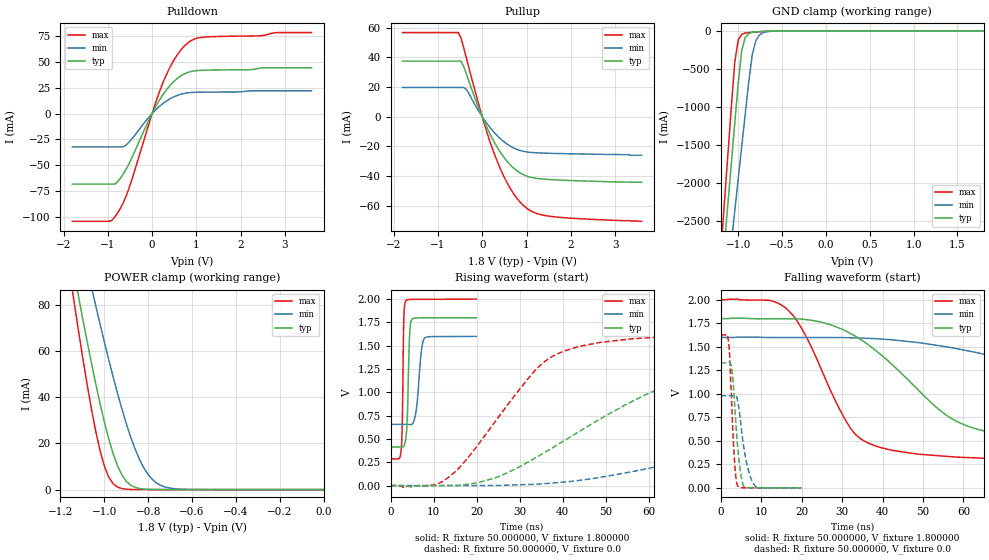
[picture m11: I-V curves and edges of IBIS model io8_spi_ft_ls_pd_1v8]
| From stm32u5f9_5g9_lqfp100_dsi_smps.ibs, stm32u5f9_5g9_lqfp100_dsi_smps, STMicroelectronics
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|   Model io8_spi_ft_ls_pd_1v8
[Model]  io8_spi_ft_ls_pd_1v8
Model_type I/O
Polarity   Non-Inverting
Enable   Active-Low
Vinl =   0.540000V
Vinh =   1.260000V
Vmeas =  0.900000V
Cref =   50.000000pF
Rref =   100.000000M
Vref =   0.0V
C_comp   3.338500pF   3.332300pF   3.378900pF
[Temperature Range]   25.000000   0.140000k   -40.000000
[Pullup Reference]   1.800000V   1.600000V   2.000000V
[Pulldown Reference]   0.0V   0.0V   0.0V
[POWER Clamp Reference]   1.800000V   1.600000V   2.000000V
[GND Clamp Reference]   0.0V   0.0V   0.0V
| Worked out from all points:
|   slope of the pulldown table from 0 to 0.27 V, typ, clamps not added: 13.6 ohm
|   slope of the pullup table from 0 to 0.27 V, typ, clamps not added: 15.9 ohm
|   GND clamp passes 1 mA (typ) near -0.50 V on its own axis
|   POWER clamp passes 1 mA (typ) near -0.86 V on its own axis
|   rising waveform, R_fixture 50.000000, V_fixture 1.800000: 20-80 % time 490ps typ, 1.02ns min, 316ps max; typ from 0.414 V to 1.8 V
|   rising waveform, R_fixture 50.000000, V_fixture 0.0: 20-80 % time 31.5ns typ, 69.2ns min, 16.6ns max; typ from 0 V to 1.33 V
|   falling waveform, R_fixture 50.000000, V_fixture 1.800000: 20-80 % time 22.7ns typ, 57.7ns min, 11.6ns max; typ from 1.8 V to 0.414 V
|   falling waveform, R_fixture 50.000000, V_fixture 0.0: 20-80 % time 1.42ns typ, 2.11ns min, 1.03ns max; typ from 1.33 V to 0 V
[Pulldown]
|Voltage   I(typ)   I(min)   I(max)
-1.8V     -68.38mA   -32.32mA   -104.4mA
-960mV    -68.38mA   -32.32mA   -104.4mA
-780mV    -66.07mA   -32.32mA   -96.42mA
-660mV    -59.2mA    -32.31mA   -87.22mA
-540mV    -50.22mA   -28.51mA   -74.66mA
0V        -10fA      -300fA     0A
240mV     18.04mA    9.599mA    29.41mA
480mV     30.68mA    16.02mA    50.95mA
780mV     39.47mA    19.98mA    67.56mA
960mV     41.44mA    20.62mA    72.37mA
1.14V     41.99mA    20.78mA    74.01mA
3.6V      44.44mA    22.06mA    78.55mA
[Pullup]
|Voltage   I(typ)   I(min)   I(max)
-1.8V     37.47mA    19.74mA    56.73mA
-540mV    37.47mA    19.74mA    56.73mA
-480mV    37.47mA    19.74mA    53.05mA
-360mV    28.94mA    18.47mA    39.74mA
0V        0A         0A         0A
300mV     -18.63mA   -11.6mA    -27.18mA
600mV     -31.41mA   -19.24mA   -46.67mA
780mV     -36.41mA   -22mA      -54.89mA
960mV     -39.54mA   -23.52mA   -60.64mA
1.2V      -41.44mA   -24.28mA   -64.93mA
1.56V     -42.42mA   -24.69mA   -67.24mA
3.6V      -44.2mA    -26mA      -70.5mA
[GND_clamp]
|Voltage   I(typ)   I(min)   I(max)
-1.8V     -9.908A    -9.683A    -9.994A
-1.2V     -3.383A    -4.084A    -2.934A
-1.16V    -2.841A    -3.655A    -2.294A
-1.12V    -2.299A    -3.226A    -1.656A
-1.04V    -1.218A    -2.369A    -414.2mA
-1V       -684.7mA   -1.941A    -119.2mA
-960mV    -257.2mA   -1.514A    -45.67mA
-920mV    -87.04mA   -1.089A    -28.94mA
-840mV    -19.36mA   -312.8mA   -18.98mA
-800mV    -13.56mA   -132.4mA   -15.51mA
-720mV    -8.053mA   -25.67mA   -9.504mA
1.8V      45.71uA    33.32uA    56.11uA
[POWER_clamp]
|Voltage   I(typ)   I(min)   I(max)
-1.8V     470.8mA    433.7mA    554.6mA
-1.14V    95.25mA    122.7mA    82.82mA
-1.12V    84.97mA    114mA      70.27mA
-1.06V    55.51mA    88.42mA    35.67mA
-1.04V    46.34mA    80.15mA    25.76mA
-1V       29.51mA    64.13mA    10.3mA
-940mV    10.39mA    41.86mA    1.109mA
-900mV    3.624mA    28.77mA    182.8uA
-840mV    490.7uA    13.24mA    11.35uA
-800mV    116.8uA    6.532mA    1.77uA
-740mV    13.2uA     1.724mA    109.3nA
0V        0A         18.75nA    0A
[Ramp]
| variable   typ   min   max
dV/dt_r  0.79740/31.46874n   0.58757/69.17353n   0.97632/16.62048n
dV/dt_f  0.83141/22.62142n   0.56503/57.71490n   1.02743/11.62477n
R_load = 50.000000
[Rising Waveform]
R_fixture= 50.000000
V_fixture= 1.800000
V_fixture_min= 1.600000
V_fixture_max= 2.000000
|time   V(typ)   V(min)   V(max)
0s        413.8mV    656.5mV    287.1mV
2.482ns   413.2mV    656.5mV    390.5mV
2.723ns   412.3mV    656.5mV    688mV
3.083ns   422.3mV    656.5mV    1.797V
3.483ns   489.6mV    656.5mV    1.977V
3.884ns   717.1mV    656.3mV    1.992V
4.444ns   1.624V     654.6mV    1.996V
4.925ns   1.779V     656.3mV    1.997V
7.808ns   1.799V     1.576V     1.998V
19.94ns   1.8V       1.599V     2V
[Rising Waveform]
R_fixture= 50.000000
V_fixture= 0.0
V_fixture_min= 0.0
V_fixture_max= 0.0
|time   V(typ)   V(min)   V(max)
0s        1.796nV    144.1nV    1.167nV
9.61ns    -441.1uV   -891.2uV   3.861mV
14.41ns   1.306mV    -187.6uV   123.8mV
24.82ns   91.01mV    1.249mV    717.8mV
36.84ns   382.2mV    24.07mV    1.363V
56.06ns   900.3mV    148.4mV    1.573V
83.28ns   1.233V     414.4mV    1.618V
121.7ns   1.31V      734mV      1.627V
157ns     1.324V     881.8mV    1.627V
398.8ns   1.329V     979.8mV    1.627V
[Falling Waveform]
R_fixture= 50.000000
V_fixture= 1.800000
V_fixture_min= 1.600000
V_fixture_max= 2.000000
|time   V(typ)   V(min)   V(max)
0s        1.8V       1.599V     2V
16.02ns   1.798V     1.598V     1.915V
20.82ns   1.791V     1.598V     1.634V
32.83ns   1.624V     1.595V     591.6mV
48.85ns   1.039V     1.545V     358mV
58.46ns   703.7mV    1.479V     326.6mV
71.27ns   555.2mV    1.357V     307.6mV
110.5ns   448.4mV    919.9mV    290.2mV
145.7ns   425.6mV    770.6mV    287.8mV
398.8ns   413.8mV    656.5mV    287.1mV
[Falling Waveform]
R_fixture= 50.000000
V_fixture= 0.0
V_fixture_min= 0.0
V_fixture_max= 0.0
|time   V(typ)   V(min)   V(max)
0s        1.329V     979.8mV    1.627V
1.562ns   1.329V     979.8mV    1.63V
2.002ns   1.332V     979.8mV    1.53V
2.763ns   1.256V     979.6mV    854.2mV
3.323ns   963.7mV    986.1mV    349mV
4.164ns   450mV      928.3mV    24.42mV
5.526ns   35.4mV     483.6mV    1.422mV
6.727ns   2.507mV    208.5mV    294.1uV
8.368ns   466.3uV    25.48mV    58.56uV
19.94ns   1.796nV    144.1nV    1.167nV
